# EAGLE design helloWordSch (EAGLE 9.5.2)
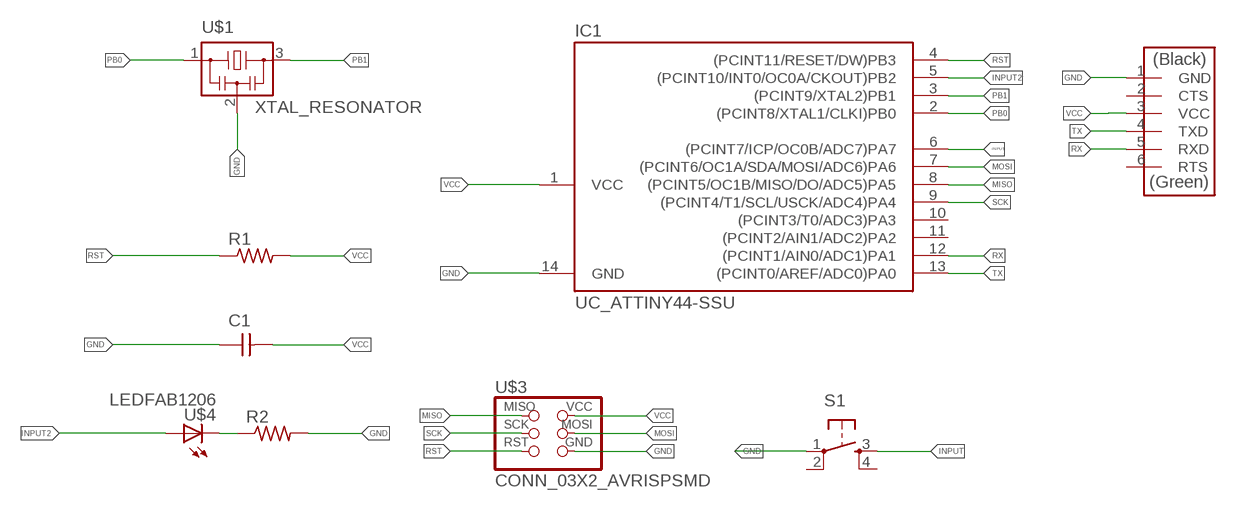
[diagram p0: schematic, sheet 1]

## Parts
C1  CAP_UNPOLARIZEDFAB  [C1206FAB]
IC1  UC_ATTINY44-SSU  [SOIC14]
R1  R1206FAB  [R1206FAB]
R2  R1206FAB  [R1206FAB]
S1  SW_SWITCH_TACTILE_6MM6MM_SWITCH  [6MM_SWITCH]
U$1  XTAL_RESONATOR  [EFOBM]
U$2  CONN_06_FTDI-SMD-HEADER  [1X06SMD]
U$3  CONN_03X2_AVRISPSMD  [2X03SMD]
U$4  LEDFAB1206  [LED1206FAB]

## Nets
GND: C1.1 IC1.14(GND) R2.2 S1.1(P) U$1.2 U$2.1(GND) U$3.6(GND)
INPUT: IC1.6((PCINT7/ICP/OC0B/ADC7)PA7) S1.3(S)
INPUT2: IC1.5((PCINT10/INT0/OC0A/CKOUT)PB2) U$4.1(A)
MISO: IC1.8((PCINT5/OC1B/MISO/DO/ADC5)PA5) U$3.1(MISO)
MOSI: IC1.7((PCINT6/OC1A/SDA/MOSI/ADC6)PA6) U$3.4(MOSI)
N$3: R2.1 U$4.2(C)
PB0: IC1.2((PCINT8/XTAL1/CLKI)PB0) U$1.1
PB1: IC1.3((PCINT9/XTAL2)PB1) U$1.3
RST: IC1.4((PCINT11/RESET/DW)PB3) R1.1 U$3.5(RST)
RX: IC1.12((PCINT1/AIN0/ADC1)PA1) U$2.5(RXD)
SCK: IC1.9((PCINT4/T1/SCL/USCK/ADC4)PA4) U$3.3(SCK)
TX: IC1.13((PCINT0/AREF/ADC0)PA0) U$2.4(TXD)
VCC: C1.2 IC1.1(VCC) R1.2 U$2.3(VCC) U$3.2(VCC)
Unconnected: IC1.10((PCINT3/T0/ADC3)PA3) IC1.11((PCINT2/AIN1/ADC2)PA2) S1.2(P1) S1.4(S1) U$2.2(CTS) U$2.6(RTS)

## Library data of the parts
C1 = eagle_fab:CAP_UNPOLARIZED
IC1 = eagle_fab:UC_ATTINY44
R1 R2 = eagle_fab:R: Resistor (US Symbol)
S1 = eagle_fab:SW_SWITCH_TACTILE_6MM: OMRON SWITCH
U$1 = eagle_fab:XTAL_RESONATOR
U$2 = eagle_fab:CONN_06_FTDI-SMD-HEADER
U$3 = eagle_fab:CONN_03X2_AVRISP
U$4 = eagle_fab:LED: LED

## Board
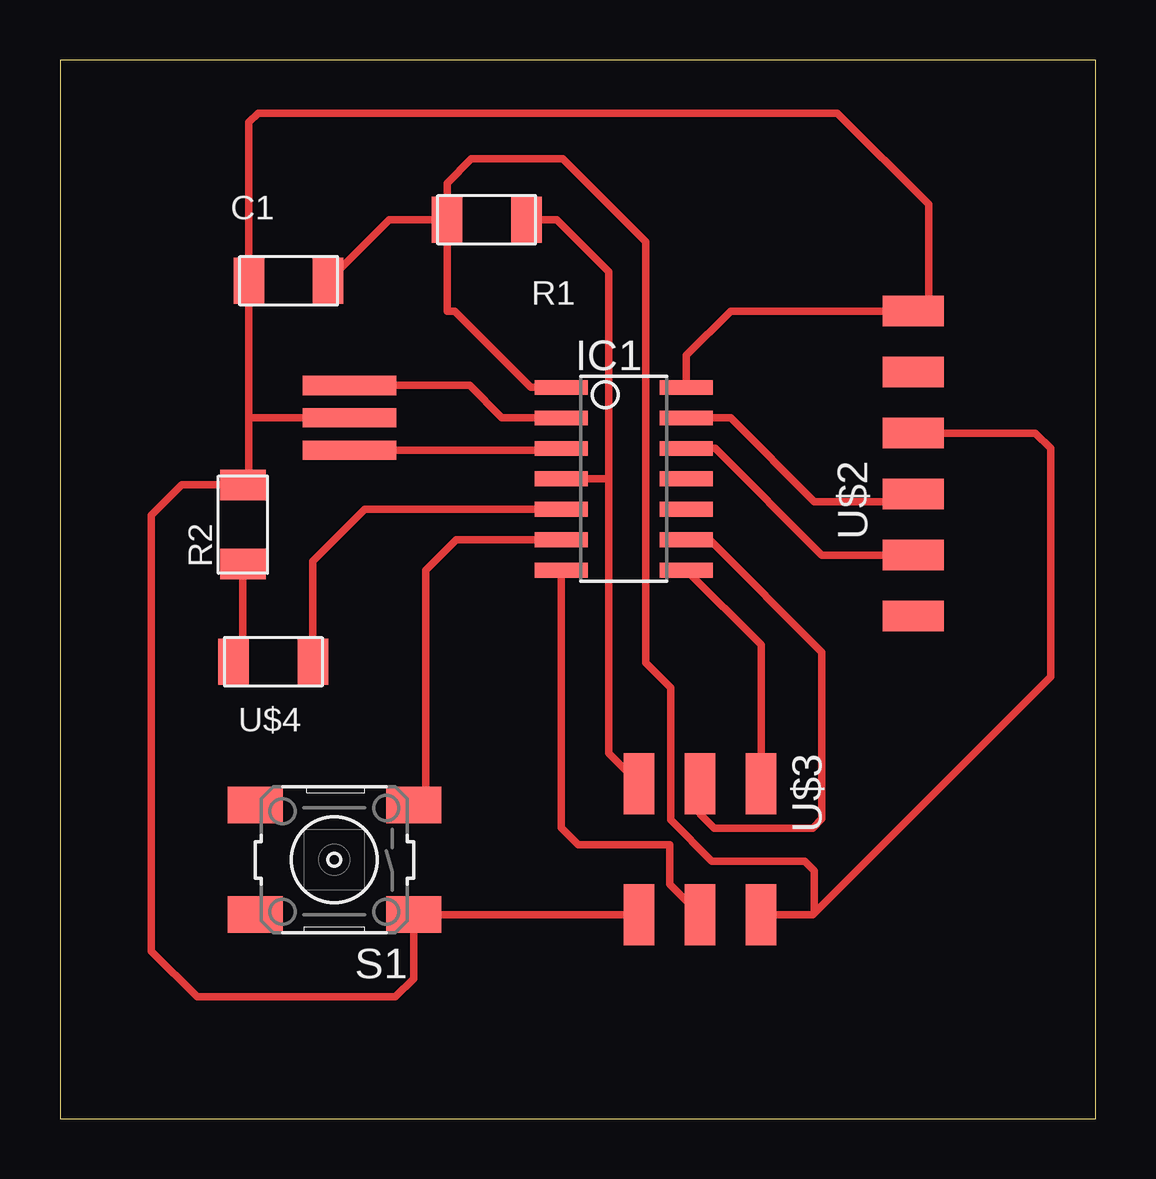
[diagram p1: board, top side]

Size 43.16 x 44.12 mm. Coordinates in mm from the lower left corner, seen from the top.
Outline: 0,0 43.16,0 43.16,44.12 0,44.12 0,0
Copper layers (1*16): Top 0.035mm / dielectric 1.5mm / Bottom 0.035mm
Design rules "default *": minimum track width 12mil, minimum drill 0.35mm, track to track 17mil, track to pad 17mil, pad to pad 17mil, via to via 17mil, smd to smd 17mil, copper to edge 40mil, drill to drill 6mil, minimum pad ring 10mil, minimum via ring 8mil, stop-mask expansion 4mil, vias tented up to drill 0mil, thermal gap 10mil

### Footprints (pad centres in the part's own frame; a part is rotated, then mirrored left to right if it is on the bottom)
C1206FAB = smd 1.27 x 1.905: 1 -1.651,0; 2 1.651,0
SOIC14 = smd 0.61 x 2.21: 1 -3.81,-2.603; 2 -2.54,-2.603; 3 -1.27,-2.603; 4 0,-2.603; 5 1.27,-2.603; 6 2.54,-2.603; 7 3.81,-2.603; 8 3.81,2.603; 9 2.54,2.603; 10 1.27,2.603; 11 0,2.603; 12 -1.27,2.603; 13 -2.54,2.603; 14 -3.81,2.603
R1206FAB = smd 1.27 x 1.905: 1 -1.651,0; 2 1.651,0
6MM_SWITCH = smd 2.286 x 1.524: 1 -3.302,2.286; 2 3.302,2.286; 3 -3.302,-2.286; 4 3.302,-2.286
EFOBM = smd 0.8 x 3.9: 1 -1.35,0; 2 0,0; 3 1.35,0
1X06SMD = smd 2.54 x 1.27: 1 0,6.35; 2 0,3.81; 3 0,1.27; 4 0,-1.27; 5 0,-3.81; 6 0,-6.35
2X03SMD = smd 2.54 x 1.27: 1 -2.54,2.54; 2 2.92,2.54; 3 -2.54,0; 4 2.92,0; 5 -2.54,-2.54; 6 2.92,-2.54
LED1206FAB = smd 1.27 x 1.905: 1 -1.651,0; 2 1.651,0

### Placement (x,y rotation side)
C1  9.52,34.92 0 top
IC1  23.49,26.67 270 top
R1  17.78,37.47 180 top
R2  7.62,24.77 90 top
S1  11.43,10.8 180 top
U$1  12.06,29.21 270 top
U$2  35.56,27.3 0 top
U$3  26.67,11.43 270 top
U$4  8.89,19.05 180 top

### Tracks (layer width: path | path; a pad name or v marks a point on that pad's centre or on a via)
GND
  Top 0.305: 7.87,29.21 C1.1 7.87,41.53 8.25,41.91 32.38,41.91 36.2,38.1 36.2,33.66 U$2.1 27.94,33.66 26.1,31.81 IC1.14 | 10.79,29.21 U$1.2 7.87,29.21 | U$3.6 S1.1 14.73,5.84 13.97,5.08 5.71,5.08 3.81,6.98 3.81,25.15 5.08,26.42 R2.2 7.87,26.67 7.87,29.21
INPUT
  Top 0.305: 20.85,24.17 IC1.6 16.51,24.13 15.24,22.86 15.24,13.59 S1.3
INPUT2
  Top 0.305: IC1.5 12.7,25.4 10.54,23.24 U$4.1
MISO
  Top 0.305: 26.04,22.8 IC1.8 29.21,19.75 U$3.1
MOSI
  Top 0.305: IC1.7 20.89,12.13 21.59,11.43 25.4,11.43 25.4,9.78 U$3.4 26.93,8.51
N$3
  Top 0.305: 7.62,22.48 R2.1 7.62,18.41 7.24,18.8 U$4.2
PB0
  Top 0.305: U$1.1 17.06,30.56 18.41,29.21 IC1.2 20.32,29.21
PB1
  Top 0.305: U$1.3 20.81,27.86 IC1.3
RST
  Top 0.305: 24.13,13.34 U$3.5 22.86,15.24 22.86,26.67 | 22.86,26.67 22.86,35.31 20.7,37.47 R1.1 | IC1.4 22.86,26.67
RX
  Top 0.305: 36.2,23.49 U$2.5 31.75,23.49 27.3,27.94 IC1.12
SCK
  Top 0.305: 26.95,14.25 U$3.3 26.67,12.7 27.25,12.12 31.36,12.12 31.75,12.51 31.75,19.44 27.06,24.13 IC1.9
TX
  Top 0.305: U$2.4 35.88,25.72 31.43,25.72 27.94,29.21 IC1.13
VCC
  Top 0.305: 29.21,7.62 U$3.2 31.37,8.51 31.43,8.57 | 31.43,8.57 41.27,18.41 41.27,27.94 40.64,28.57 U$2.3 35.61,28.52 | R1.2 13.72,37.47 C1.2 | R1.2 16.13,33.66 16.45,33.66 19.62,30.48 IC1.1 | R1.2 16.13,38.99 17.14,40 20.95,40 24.41,36.55 24.41,19 25.45,17.96 25.45,12.46 27.16,10.74 31.03,10.74 31.43,10.34 31.43,8.57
